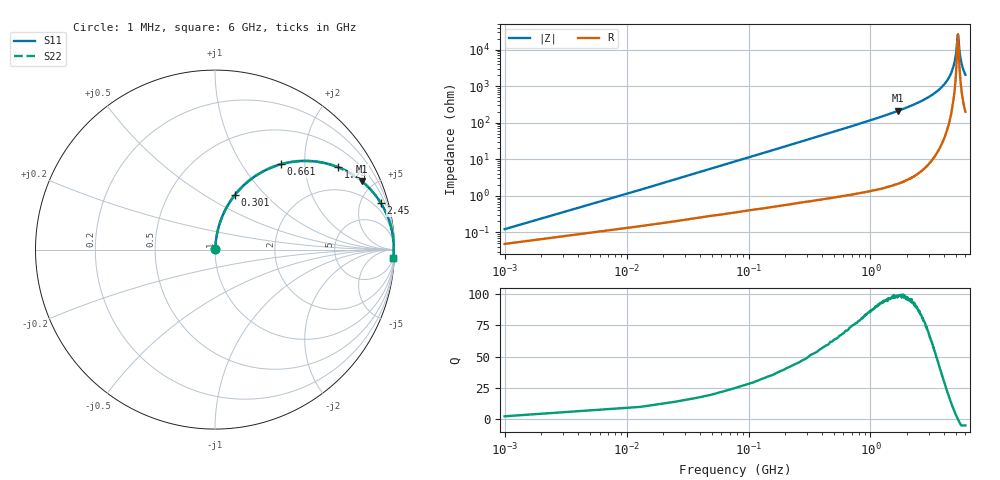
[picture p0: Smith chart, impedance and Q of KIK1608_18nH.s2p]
!version-2
!date-01.2022
!Series
# MHz S RI R 50
!Freq ReS11 ImS11 ReS21 ImS21 ReS12 ImS12 ReS22 ImS22
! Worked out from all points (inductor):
!   501 points, 1 MHz to 6 GHz, reference 50 ohm
!   read as one part in series: L = 18 nH near 25 MHz
!   highest Q = 98.7 at 1.69 GHz (marker M1), where L = 20.2 nH
!   self-resonance near 5.21 GHz
!   S11 on the Smith chart (normalised r, x): 1 MHz: 1.00, +0.00; 301 MHz: 1.01, +0.68; 661 MHz: 1.02, +1.52; 1.24 GHz: 1.03, +2.97; 2.45 GHz: 1.08, +7.11; 6 GHz: 5, -41
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1  0.000475 0.00113  0.9995 -0.00113  0.9995 -0.00113  0.000475 0.00113
37  0.0042 0.0416  0.9958 -0.0416  0.9958 -0.0416  0.0042 0.0416
73  0.0101 0.0815  0.9899 -0.0815  0.9899 -0.0815  0.0101 0.0815
157  0.0352 0.1706  0.9648 -0.1706  0.9648 -0.1706  0.0352 0.1706
301  0.1094 0.3021  0.8906 -0.3021  0.8906 -0.3021  0.1094 0.3021
661  0.3678 0.4753  0.6322 -0.4753  0.6322 -0.4753  0.3678 0.4753
1010  0.5834 0.4873  0.4166 -0.4873  0.4166 -0.4873  0.5834 0.4873
1240  0.6855 0.459  0.3145 -0.459  0.3145 -0.459  0.6855 0.459
1690  0.8184 0.3805  0.1816 -0.3805  0.1816 -0.3805  0.8184 0.3805
2020  0.8755 0.325  0.1245 -0.325  0.1245 -0.325  0.8755 0.325
2450  0.9242 0.2591  0.0758 -0.2591  0.0758 -0.2591  0.9242 0.2591
3010  0.9607 0.1871  0.0393 -0.1871  0.0393 -0.1871  0.9607 0.1871
4010  0.9891 0.0887  0.0109 -0.0887  0.0109 -0.0887  0.9891 0.0887
4660  0.9952 0.0379  0.0048 -0.0379  0.0048 -0.0379  0.9952 0.0379
5010  0.9962 0.0136  0.00382 -0.0136  0.00382 -0.0136  0.9962 0.0136
5170  0.9962 0.00244  0.00379 -0.00244  0.00379 -0.00244  0.9962 0.00244
5210  0.9962 0.000105  0.00381 -0.000105  0.00381 -0.000105  0.9962 0.000105
5260  0.9961 -0.00298  0.00386 0.00298  0.00386 0.00298  0.9961 -0.00298
5360  0.9959 -0.00983  0.00406 0.00983  0.00406 0.00983  0.9959 -0.00983
5480  0.9956 -0.0173  0.00438 0.0173  0.00438 0.0173  0.9956 -0.0173
5710  0.9947 -0.031  0.00528 0.031  0.00528 0.031  0.9947 -0.031
6000  0.9931 -0.0475  0.0069 0.0475  0.0069 0.0475  0.9931 -0.0475
